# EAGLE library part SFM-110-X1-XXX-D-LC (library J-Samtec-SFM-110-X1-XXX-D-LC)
0.05"X0.05" SOCKET STRIP DOUBLE ROW ASSEMBLY. MANUFACTURER: SAMTEC.
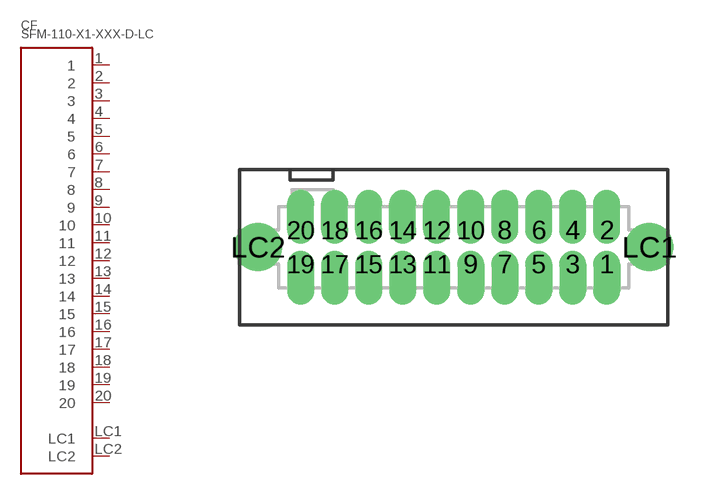
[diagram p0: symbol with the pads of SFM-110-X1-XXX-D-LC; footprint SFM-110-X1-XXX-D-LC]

Designator prefix CF

## SFM-110-X1-XXX-D-LC  [SFM-110-X1-XXX-D-LC]
1  1  pas
2  2  pas
3  3  pas
4  4  pas
5  5  pas
6  6  pas
7  7  pas
8  8  pas
9  9  pas
10  10  pas
11  11  pas
12  12  pas
13  13  pas
14  14  pas
15  15  pas
16  16  pas
17  17  pas
18  18  pas
19  19  pas
20  20  pas
LC1  LC1  pas
LC2  LC2  pas

## Footprint SFM-110-X1-XXX-D-LC (pad centres in mm)
0.05"X0.05" SOCKET STRIP DOUBLE ROW ASSEMBLY. MANUFACTURER: SAMTEC.
drill 0.5 offset: 1 5.715,-0.635; 2 5.715,0.635; 3 4.445,-0.635; 4 4.445,0.635; 5 3.175,-0.635; 6 3.175,0.635; 7 1.905,-0.635; 8 1.905,0.635; 9 0.635,-0.635; 10 0.635,0.635; 11 -0.635,-0.635; 12 -0.635,0.635; 13 -1.905,-0.635; 14 -1.905,0.635; 15 -3.175,-0.635; 16 -3.175,0.635; 17 -4.445,-0.635; 18 -4.445,0.635; 19 -5.715,-0.635; 20 -5.715,0.635
drill 1.194: LC1 7.303,0; LC2 -7.303,0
